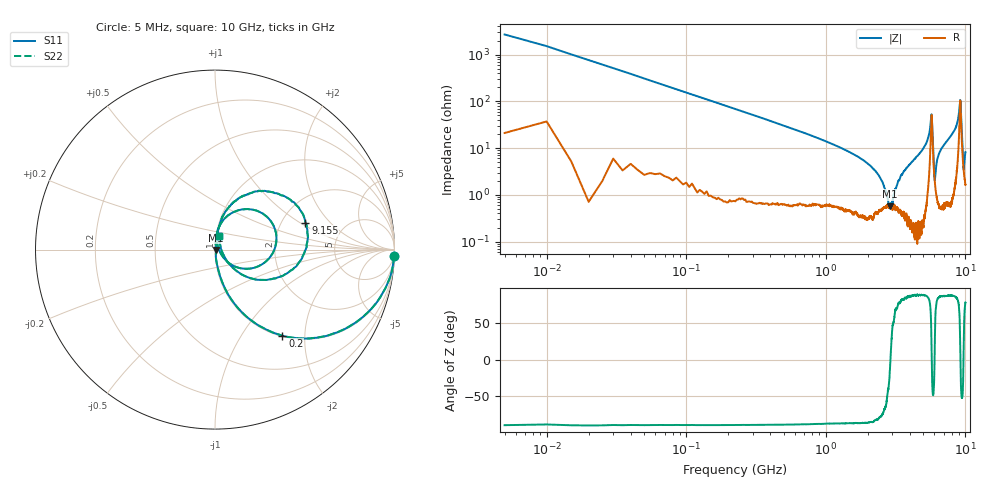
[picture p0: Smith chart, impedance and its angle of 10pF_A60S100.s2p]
! Amotech Co.,Ltd.
! http://www.amotech.co.kr/
! Part Number: A60S100
! These Parameters are Measured in Series Mode Connection
! Operation Temp=25[degC], DC Bias Voltage=0[V]
! Freq. Start=5[MHz] Stop=10[GHz], 2000[Steps]
! Date: Monday, July 13, 2020, 01:35:10
# GHZ S RI R 50.000000
!Freq.(Hz) S11(Real) S11(Imag) S21(Real) S21(Imag) S12(Real) S12(Imag) S22(Real) S22(Imag)
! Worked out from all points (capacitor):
!   2000 points, 5 MHz to 10 GHz, reference 50 ohm
!   read as one part in series: C = 10.3 pF near 55 MHz
!   lowest |Z| = 571 mohm at 2.86 GHz (marker M1)
!   series resonance near 2.904 GHz, so ESL is about 290 pH
!   S11 on the Smith chart (normalised r, x): 5 MHz: 1, -54; 200 MHz: 1.01, -1.55; 9.155 GHz: 2.70, +1.10; 10 GHz: 1.03, +0.16
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0.005  0.9983 -0.0371  0.00167 0.0371  0.00167 0.0371  0.9983 -0.0371
0.085  0.7641 -0.4182  0.2359 0.4182  0.2359 0.4182  0.7641 -0.4182
0.2  0.3754 -0.4798  0.6246 0.4798  0.6246 0.4798  0.3754 -0.4798
0.55  0.0747 -0.2525  0.9253 0.2525  0.9253 0.2525  0.0747 -0.2525
1.675  0.00847 -0.0662  0.9915 0.0662  0.9915 0.0662  0.00847 -0.0662
2.405  0.00506 -0.0251  0.9949 0.0251  0.9949 0.0251  0.00506 -0.0251
2.86  0.00519 -0.00232  0.9948 0.00232  0.9948 0.00232  0.00519 -0.00232
3.34  0.00495 0.0201  0.9951 -0.0201  0.9951 -0.0201  0.00495 0.0201
5.005  0.0118 0.098  0.9882 -0.098  0.9882 -0.098  0.0118 0.098
5.505  0.0634 0.1824  0.9366 -0.1824  0.9366 -0.1824  0.0634 0.1824
5.715  0.3398 0.0929  0.6602 -0.0929  0.6602 -0.0929  0.3398 0.0929
5.81  0.1569 -0.1058  0.8431 0.1058  0.8431 0.1058  0.1569 -0.1058
5.98  0.0264 -0.012  0.9736 0.012  0.9736 0.012  0.0264 -0.012
6.04  0.0182 0.00765  0.9818 -0.00765  0.9818 -0.00765  0.0182 0.00765
6.295  0.0108 0.057  0.9892 -0.057  0.9892 -0.057  0.0108 0.057
6.67  0.0136 0.0902  0.9864 -0.0902  0.9864 -0.0902  0.0136 0.0902
8.335  0.0639 0.2197  0.9361 -0.2197  0.9361 -0.2197  0.0639 0.2197
8.97  0.269 0.3265  0.731 -0.3265  0.731 -0.3265  0.269 0.3265
9.155  0.5036 0.1479  0.4964 -0.1479  0.4964 -0.1479  0.5036 0.1479
9.33  0.2865 -0.1692  0.7135 0.1692  0.7135 0.1692  0.2865 -0.1692
9.7  0.0343 0.000755  0.9657 -0.000755  0.9657 -0.000755  0.0343 0.000755
10  0.0223 0.078  0.9777 -0.078  0.9777 -0.078  0.0223 0.078
